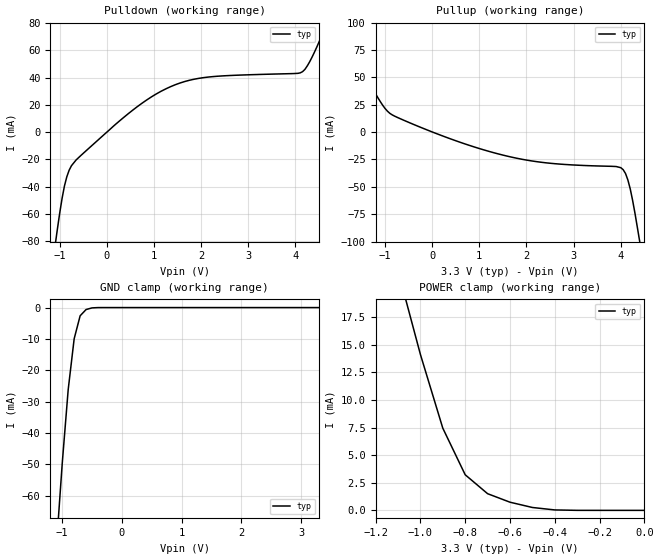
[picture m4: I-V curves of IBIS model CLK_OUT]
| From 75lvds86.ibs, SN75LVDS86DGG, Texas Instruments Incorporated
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|   Receiver Clock Output  MODEL
[Model]   CLK_OUT
Model_type   3-state
| Signals   CLKOUT
Vmeas = 1.5V   |Reference voltage for timing measurements
Cref = 8pF   |Timing specification test load capacitance value
Vref = 0   |Timing specification test load voltage; GND
| variable   typ   min   max
C_comp   1.0pF   NA   NA
|   typ   min   max
[Temperature Range]   25.0   NA   NA
[Voltage range]   3.3V   3.0V   3.6V
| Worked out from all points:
|   slope of the pulldown table from 0 to 0.495 V, typ, clamps not added: 33.8 ohm
|   slope of the pullup table from 0 to 0.495 V, typ, clamps not added: 62.3 ohm
|   GND clamp passes 1 mA (typ) near -0.62 V on its own axis
|   POWER clamp passes 1 mA (typ) near -0.63 V on its own axis
[Pulldown]
|   Voltage   I(typ)   I(min)   I(max)
-3.3V     -629.8mA   NA         NA
-1.1V     -83.77mA   NA         NA
-1.05V    -71.36mA   NA         NA
-900mV    -39.59mA   NA         NA
-750mV    -24.61mA   NA         NA
450mV     13.38mA    NA         NA
1.35V     33.29mA    NA         NA
2.15V     40.35mA    NA         NA
4.1V      43.42mA    NA         NA
4.25V     48.53mA    NA         NA
4.5V      66.15mA    NA         NA
6.6V      231.7mA    NA         NA
[Pullup]
|   Voltage   I(typ)   I(min)   I(max)
| Note that the[Pullup]voltage table is referenced to Vcc
| and is calculated using Vtable=Vcc - Vmeasured.
-3.3V     188.7mA    NA         NA
-1.2V     34.95mA    NA         NA
-900mV    17.2mA     NA         NA
-300mV    5.322mA    NA         NA
800mV     -12.3mA    NA         NA
1.8V      -23.95mA   NA         NA
4V        -32.53mA   NA         NA
4.1V      -37.83mA   NA         NA
4.15V     -43.73mA   NA         NA
4.25V     -62.28mA   NA         NA
4.4V      -99.75mA   NA         NA
6.6V      -670.4mA   NA         NA
[GND_clamp]
|   Voltage   I(typ)   I(min)   I(max)
| Outputs in Tri-state.
-3.3V     -740mA     NA         NA
-1.1V     -76.92mA   NA         NA
-1V       -49.78mA   NA         NA
-900mV    -26.17mA   NA         NA
-800mV    -9.95mA    NA         NA
-700mV    -2.62mA    NA         NA
-600mV    -620uA     NA         NA
-500mV    -100uA     NA         NA
-400mV    -5.98uA    NA         NA
3.3V      350pA      NA         NA
[POWER_clamp]
|   Voltage   I(typ)   I(min)   I(max)
| Note that the [POWER_clamp] voltage table is referenced to Vcc
| and is calculated using Vtable = Vcc - Vmeasured.
| Outputs in Tri-state.
-3.3V     208.5mA    NA         NA
-1.1V     21.72mA    NA         NA
-1V       14.13mA    NA         NA
-900mV    7.445mA    NA         NA
-800mV    3.224mA    NA         NA
-700mV    1.51mA     NA         NA
-600mV    739uA      NA         NA
-500mV    260uA      NA         NA
-400mV    38.9uA     NA         NA
0V        -9.18nA    NA         NA
[Ramp]
|   typ   min   max
dV/dt_r   1.903v/533ps   NA   NA
dV/dt_f   1.922v/565ps   NA   NA
R_load = 1000ohm
